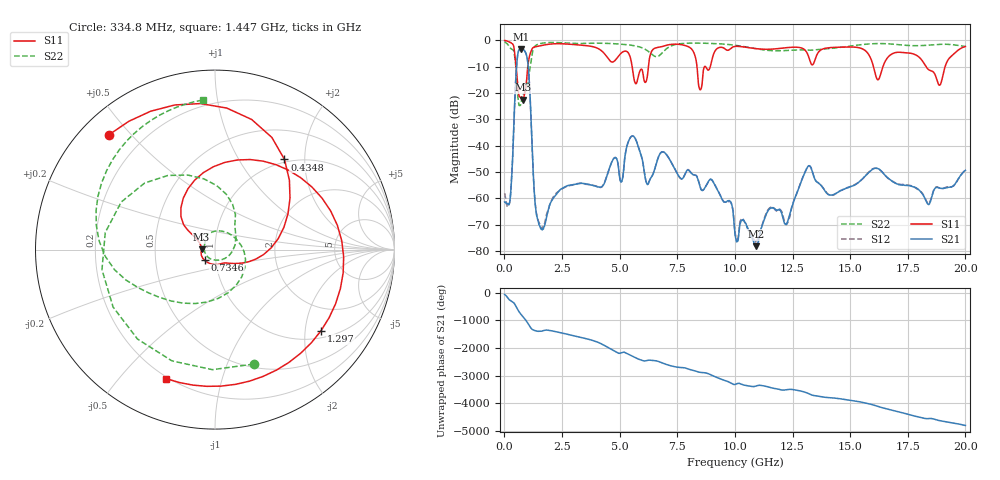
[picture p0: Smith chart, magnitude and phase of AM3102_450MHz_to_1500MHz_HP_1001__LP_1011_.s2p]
!Agilent Technologies,E8364B,MY43040894,A.07.50.67
!Agilent E8364B: A.07.50.67
!Date: Thursday, January 11, 2018 06:04:15
!Correction: S11(Full 2 Port(1,2))
!S21(Full 2 Port(1,2))
!S12(Full 2 Port(1,2))
!S22(Full 2 Port(1,2))
!S2P File: Measurements: S11, S21, S12, S22:
# Hz S  dB  R 50
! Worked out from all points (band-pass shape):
!   1601 points, 10 MHz to 20 GHz, reference 50 ohm
!   highest |S21| = -3.24 dB at 734.6 MHz (marker M1); lowest = -78.1 dB at 10.93 GHz (marker M2)
!   |S21| within 3 dB of the highest: 567.4 MHz to 976.6 MHz (409.2 MHz wide, 53 % of centre)
!   lowest |S11| = -22.5 dB at 797.1 MHz (marker M3), VSWR 1.16, Z = 43 + j0.192 ohm
!   |S11| at or under -10 dB: 508.9 MHz to 1.015 GHz (506.1 MHz wide, 66.4 % of centre); 5.543 GHz to 6.248 GHz (704.9 MHz wide, 12 % of centre); 18.29 GHz to 19.12 GHz (825.4 MHz wide, 4.41 % of centre)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
!   |S22| runs from -24.8 to -0.6 dB; largest |S21 - S12| = 0.0014
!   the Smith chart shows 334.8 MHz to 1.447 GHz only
!   S11 on the Smith chart (normalised r, x): 334.8 MHz: 0.08, +0.44; 434.8 MHz: 0.95, +1.60; 734.6 MHz: 0.88, -0.11; 1.297 GHz: 1.20, -2.43; 1.447 GHz: 0.19, -0.67
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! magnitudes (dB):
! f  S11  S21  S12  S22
! 10 MHz  -0.1  -61.3  -58.0  -0.6
! 197.4 MHz  -0.6  -62.4  -61.9  -2.1
! 334.8 MHz  -1.2  -49.1  -48.9  -3.4
! 434.8 MHz  -4.0  -26.3  -26.3  -5.4
! 734.6 MHz  -21.6  -3.2  -3.2  -23.3
! 797.1 MHz  -22.5  -3.4  -3.4  -20.4
! 1.034 GHz  -8.6  -9.9  -9.9  -15.0
! 1.297 GHz  -2.6  -57.5  -57.5  -2.5
! 1.447 GHz  -2.3  -68.1  -67.9  -1.6
! 3.346 GHz  -1.9  -54.3  -54.2  -1.2
! 5.082 GHz  -4.8  -53.7  -53.6  -1.5
! 5.707 GHz  -16.5  -37.8  -37.8  -2.2
! 6.207 GHz  -13.4  -54.7  -54.6  -4.0
! 6.682 GHz  -2.7  -44.3  -44.3  -6.0
! 8.081 GHz  -3.0  -50.1  -50.0  -1.1
! 8.493 GHz  -18.8  -55.7  -55.5  -1.1
! 10.01 GHz  -2.3  -73.9  -72.9  -1.9
! 10.93 GHz  -3.2  -78.1  -76.4  -3.2
! 13.34 GHz  -9.3  -49.3  -49.3  -3.7
! 16.68 GHz  -6.1  -52.5  -52.6  -1.3
! 18.88 GHz  -17.0  -56.0  -56.1  -1.5
! 20 GHz  -2.4  -49.3  -49.4  -2.3
